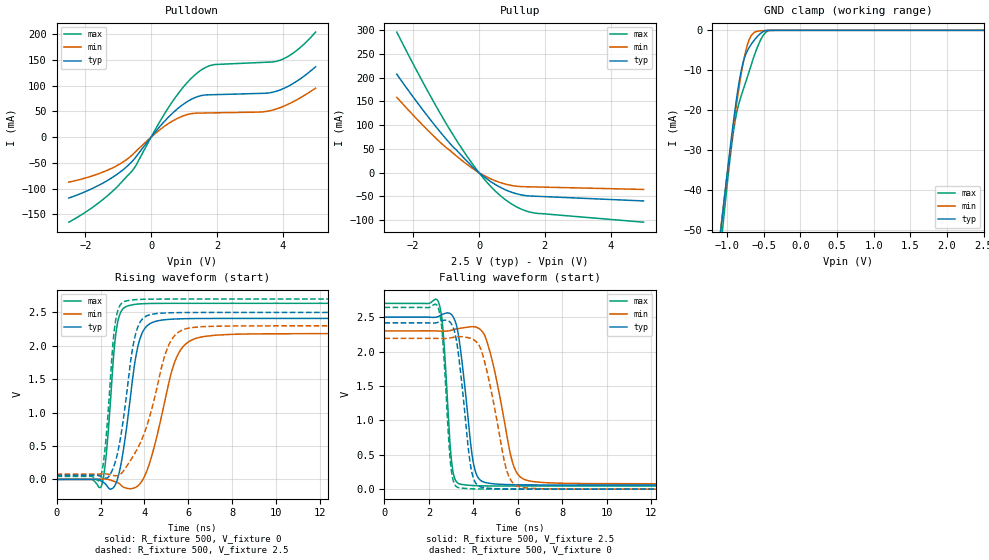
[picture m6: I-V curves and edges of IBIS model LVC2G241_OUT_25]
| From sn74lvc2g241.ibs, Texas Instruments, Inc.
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[Model]   LVC2G241_OUT_25
Model_type  3-state
Enable   Active-High
Vref =   0
Rref =   500
Cref =   30p
Vmeas =   1.25
| variable   typ   min   max
C_comp   5.97pF   5.10pF   6.99pF
| C_pullup   10.29pF   6.16pF   12.63pF
| C_pulldown   9.97pF   6.52pF   14.49pF
| C_tri-state   5.97pF   5.10pF   6.99pF
[Temperature Range]   40   100   -40
| Ambient temperature   25   85   -40
[Voltage range]   2.5   2.3   2.7
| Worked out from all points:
|   slope of the pulldown table from 0 to 0.375 V, typ, clamps not added: 13.1 ohm
|   slope of the pullup table from 0 to 0.375 V, typ, clamps not added: 19 ohm
|   GND clamp passes 1 mA (typ) near -0.56 V on its own axis
|   rising waveform, R_fixture 500, V_fixture 0: 20-80 % time 600ps typ, 961ps min, 368ps max; typ from 0 V to 2.41 V
|   falling waveform, R_fixture 500, V_fixture 2.5: 20-80 % time 494ps typ, 800ps min, 302ps max; typ from 2.5 V to 0.06 V
|   rising waveform, R_fixture 500, V_fixture 2.5: 20-80 % time 618ps typ, 1.15ns min, 366ps max; typ from 0.06 V to 2.5 V
|   falling waveform, R_fixture 500, V_fixture 0: 20-80 % time 475ps typ, 792ps min, 296ps max; typ from 2.42 V to 0 V
[GND Clamp]
| LVC2G241_OUT_25
|   Voltage   I(typ)   I(min)   I(max)
-2.5V     -315.3mA   -295.4mA   -349.7mA
-1.085V   -50.05mA   -49.49mA   -54.32mA
-1.05V    -44.23mA   -44.11mA   -47.87mA
-915mV    -23.21mA   -24.44mA   -25.71mA
-875mV    -17.74mA   -19.11mA   -21.2mA
-825mV    -11.87mA   -12.98mA   -17.5mA
-775mV    -7.672mA   -7.713mA   -14.61mA
-720mV    -5.02mA    -3.473mA   -11.53mA
-620mV    -2.264mA   -439.8uA   -5.885mA
-520mV    -448uA     -102.4uA   -1.671mA
-420mV    -4.422uA   -33.13uA   -10.75uA
2.5V      22.51pA    62.63nA    611.4pA
[Pulldown]
| LVC2G241_OUT_25
|   Voltage   I(typ)   I(min)   I(max)
-2.5V     -118.5mA   -87.61mA   -165.6mA
-1.45V    -88.91mA   -67.64mA   -120.7mA
-595mV    -48.39mA   -35.77mA   -66.9mA
125mV     10.03mA    7.029mA    14.56mA
605mV     43.82mA    29.64mA    65.06mA
1.035V    66.53mA    42.71mA    101.7mA
1.435V    79.4mA     46.8mA     126.6mA
1.91V     82.71mA    47.34mA    141.1mA
3.375V    85.29mA    49.17mA    145.5mA
3.91V     91.63mA    57.17mA    149.7mA
4.425V    108.8mA    72.58mA    168.7mA
5V        137mA      95.22mA    204.6mA
[Pullup]
| LVC2G241_OUT_25
|   Voltage   I(typ)   I(min)   I(max)
-2.5V     207.3mA    158.8mA    296.1mA
-1.96V    155.5mA    118.1mA    223.5mA
-1.47V    110.8mA    83.31mA    160.6mA
-940mV    66.09mA    50.01mA    96.79mA
-615mV    42.44mA    31.07mA    60.62mA
-250mV    16.19mA    11.66mA    23.38mA
130mV     -7.395mA   -5.203mA   -11.26mA
455mV     -23.23mA   -15.98mA   -35.95mA
780mV     -35.34mA   -23.63mA   -55.73mA
1.23V     -45.95mA   -29.05mA   -75.02mA
1.68V     -49.47mA   -29.98mA   -84.88mA
5V        -59.5mA    -35.26mA   -104.3mA
[Ramp]
| LVC2G241_OUT_25
| variable   typ   min   max
dV/dt_r   1.53/6.39E-10   1.39/1.03E-09   1.65/3.93E-10
dV/dt_f   1.50/5.14E-10   1.37/8.30E-10   1.63/3.16E-10
R_load = 500
[Rising Waveform]
| LVC2G241_OUT_25
R_fixture =   500
C_fixture =   0
L_fixture =   0
V_fixture =   0
V_fixture_min = 0
V_fixture_max = 0
|   Time   V(typ)   V(min)   V(max)
0s        123.6pV    5.829nV    2.515nV
2.035ns   -25.24mV   2.824mV    -103.1mV
2.265ns   -84.01mV   4.513mV    388.3mV
2.72ns    -44.85mV   -40.86mV   2.235V
3.27ns    991.9mV    -137mV     2.601V
3.63ns    1.88V      -112.9mV   2.623V
4.01ns    2.259V     52.59mV    2.631V
5.38ns    2.401V     1.763V     2.636V
6.33ns    2.408V     2.111V     2.637V
24.99ns   2.41V      2.183V     2.637V
[Falling Waveform]
| LVC2G241_OUT_25
R_fixture =   500
C_fixture =   0
L_fixture =   0
V_fixture =   2.5
V_fixture_min = 2.3
V_fixture_max = 2.7
|   Time   V(typ)   V(min)   V(max)
0s        2.5V       2.3V       2.7V
2.425ns   2.509V     2.297V     2.722V
2.63ns    2.542V     2.296V     2.328V
3.025ns   2.533V     2.309V     390.8mV
3.395ns   2.094V     2.337V     74.37mV
4.175ns   189.6mV    2.348V     50.05mV
4.79ns    82.32mV    1.944V     46.57mV
5.785ns   64.73mV    366.4mV    45.38mV
6.385ns   62.23mV    130.9mV    45.23mV
24.99ns   60.12mV    78.19mV    45.07mV
[Rising Waveform]
| LVC2G241_OUT_25
R_fixture =   500
C_fixture =   0
L_fixture =   0
V_fixture =   2.5
V_fixture_min = 2.3
V_fixture_max = 2.7
|   Time   V(typ)   V(min)   V(max)
0s        60.06mV    78.11mV    45.04mV
1.985ns   46.74mV    79.9mV     14.6mV
2.225ns   19.74mV    83mV       525mV
2.665ns   254.9mV    55.19mV    2.328V
3.115ns   1.088V     158.8mV    2.667V
3.475ns   1.991V     342.9mV    2.688V
3.82ns    2.365V     554.3mV    2.695V
5.035ns   2.493V     1.957V     2.7V
5.86ns    2.498V     2.253V     2.7V
24.99ns   2.5V       2.3V       2.7V
[Falling Waveform]
| LVC2G241_OUT_25
R_fixture =   500
C_fixture =   0
L_fixture =   0
V_fixture =   0
V_fixture_min = 0
V_fixture_max = 0
|   Time   V(typ)   V(min)   V(max)
0s        2.416V     2.191V     2.64V
2.405ns   2.424V     2.189V     2.649V
2.605ns   2.449V     2.188V     2.256V
2.985ns   2.413V     2.199V     337.2mV
3.315ns   1.996V     2.215V     23.53mV
4.035ns   134.1mV    2.167V     4.168mV
4.545ns   18mV       1.801V     1.399mV
5.5ns     2.974mV    272.7mV    301.2uV
6.04ns    1.312mV    38.28mV    174.7uV
24.99ns   48.11uV    67.19uV    36.21uV
